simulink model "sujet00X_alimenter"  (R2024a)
settings: Solver=FixedStepDiscrete  StartTime=0.0  StopTime=0.25  FixedStep=Ts  MaxStep=2e-6  EnableMultiTasking=on
PreLoadFcn:
  | assignin('base','Ts',1e-6);
InitFcn:
  | Ts=1e-6;
undefined symbols (not defined in the file): DiscIntNeverNeededParam, sigbuilder_block
libraries: spsUniversalBridgeLib x2, spsCurrentMeasurementLib x2, spsDCVoltageSourceLib x1, spsStepperMotorLib x1, spspowerguiLib x1

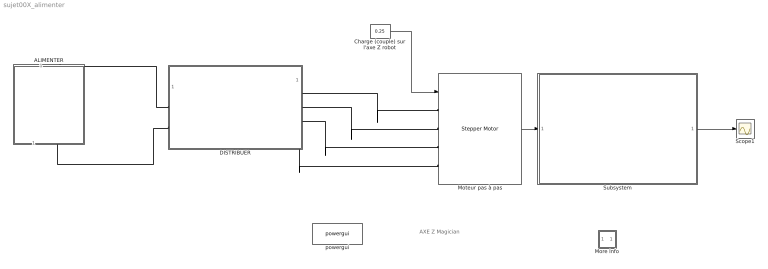
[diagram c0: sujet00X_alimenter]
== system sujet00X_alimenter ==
  note: AXE Z Magician
  ALIMENTER : Subsystem
  Charge (couple) sur l'axe Z robot : Constant  Value=0.25
  DISTRIBUER : Subsystem
  More Info : Subsystem
  Moteur pas à pas : spsStepperMotorLib/Stepper Motor  MotorType=Permanent-magnet / Hybrid  NumberOfPhases_1=2  NumberOfPhases_2=3  PresetModel_1=<empty>  PresetModel_2=<empty>  L=3e-3  Lmax=10e-3  Lmin=2e-3  R=2.1  Step_angle=1.8  Psim=0.005  Tdm=0.002  J=1.2e-7  B=1e-7*1000  w0=0  pos0=0  TsPowergui=0  TsBlock=-1
  Scope1 : Scope
  Subsystem : Subsystem
  powergui : spspowerguiLib/powergui  SimulationMode=Discrete  SampleTime=Ts  frequency=60  Iterations=50  frequencyindice=0  Pbase=100e6  ErrMax=1e-4  UnitsV=kV  UnitsW=MW  buscounter=0  FunctionMessages=off  echomessages=off  EnableUseOfTLC=off  CurrentSourceSwitches=off  DisableSnubberDevices=off  DisableRonSwitches=off  DisableVfSwitches=off  DisplayEquations=off  AutomaticDiscreteSolvers=off  SolverType=Tustin/Backward Euler (TBE)  Interpol=off  ExternalGateDelay=off  methode=off  Ts=0  x0status=blocks  SPID=off  SwTol=0  HookPort=off  NonlinearTolerance=1e-4  nMaxIteration=100  ContinueOnMaxIteration=off  RestoreLinks=warning  ResistiveCurrentMeasurement=off  Frange=[0:2:500]  Ylog=off  Xlog=on  ShowGrid=off  save=off  variable=ZData  structure=0  ZoomFFT=on  StartTime=0.0  cycles=1  DisplayStyle=1  fundamental=60  FreqAxis=off  MaxFrequency=1000  frequencyindicesteady=1  RmsSteady=1  display=off
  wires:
  Charge (couple) sur l'axe Z robot/1 -> Moteur pas à pas/1
  Moteur pas à pas/1 -> Subsystem/1(In1)
  Subsystem/1(Theta (degrees)) -> Scope1/1
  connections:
  DISTRIBUER/RConn1 -- Moteur pas à pas/LConn1
  ALIMENTER/RConn1 -- DISTRIBUER/LConn1
  DISTRIBUER/RConn2 -- Moteur pas à pas/LConn2
  DISTRIBUER/RConn3 -- Moteur pas à pas/LConn3
  DISTRIBUER/RConn4 -- Moteur pas à pas/LConn4
  DISTRIBUER/LConn2 -- ALIMENTER/LConn1

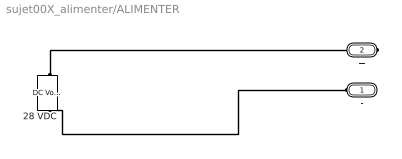
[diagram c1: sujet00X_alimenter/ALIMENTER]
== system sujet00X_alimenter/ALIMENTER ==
  28 VDC : spsDCVoltageSourceLib/DC Voltage Source  Amplitude=25.2  Measurements=None
  - : PMIOPort  Side=Left
  + : PMIOPort  Port=2  Side=Right
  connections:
  -/RConn1 -- 28 VDC/LConn1
  28 VDC/RConn1 -- +/RConn1

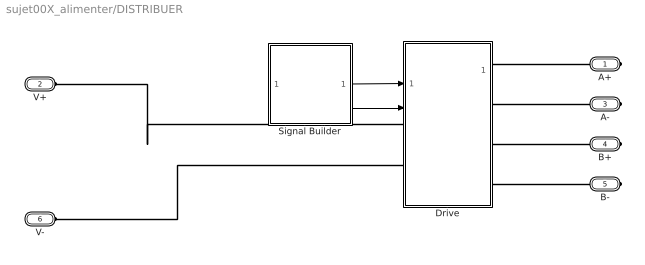
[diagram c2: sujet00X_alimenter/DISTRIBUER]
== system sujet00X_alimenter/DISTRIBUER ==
  Drive : Subsystem  mask{Iref=2, step=1200, Ts=Ts}
      mask prompts: Iref "Phase current (A)"; step "Stepping rate (step/s)"; Ts "Sampling time (s)"
      mask init:
      | Nstep=round(1/step/Ts);
  Signal Builder : Subsystem  Tag=STV Subsys  LoadFcn=sigbuilder_block('load',[90.75 199.5 600 363.75 ]);  StartFcn=sigbuilder_block('start');  StopFcn=sigbuilder_block('stop');  ClipboardFcn=sigbuilder_block('clipboard');  mask(Sigbuilder block){tuvar=[0:10]}
      mask help: Sigbuilder GUI
      mask init:
      | if ~strcmp(get_param(bdroot(gcbh),'SimulationStatus'),'stopped') tuvar = sigbuilder_block('maskInit'); end
  A+ : PMIOPort  Side=Right
  V+ : PMIOPort  Port=2  Side=Left
  A- : PMIOPort  Port=3  Side=Right
  B+ : PMIOPort  Port=4  Side=Right
  B- : PMIOPort  Port=5  Side=Right
  V- : PMIOPort  Port=6  Side=Left
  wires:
  Signal Builder/1(STEP) -> Drive/1(STEP)
  Signal Builder/2(DIR) -> Drive/2(DIR)
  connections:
  Drive/LConn2 -- V-/RConn1
  Drive/RConn4 -- B-/RConn1
  Drive/RConn1 -- A+/RConn1
  Drive/RConn2 -- A-/RConn1
  V+/RConn1 -- Drive/LConn1
  Drive/RConn3 -- B+/RConn1

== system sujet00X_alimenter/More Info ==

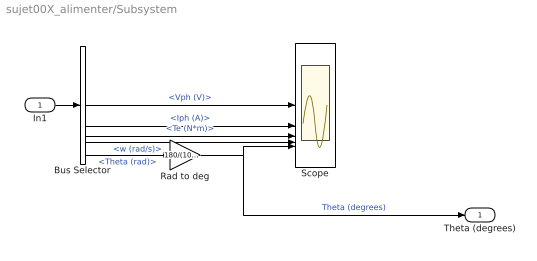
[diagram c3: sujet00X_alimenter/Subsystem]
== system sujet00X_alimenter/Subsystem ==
  In1 : Inport
  Bus Selector : BusSelector  OutputSignals=Vph (V),Iph (A),Te (N*m),w (rad/s),Theta (rad)
  Rad to deg : Gain  Gain=180/(10*pi)
  Scope : Scope  NumInputPorts=5
  Theta (degrees) : Outport
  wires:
  Rad to deg/1 -> Theta (degrees)/1, Scope/5  "Theta (degrees)"
  Bus Selector/2 -> Scope/2  "<Iph (A)>"
  Bus Selector/4 -> Scope/4  "<w (rad/s)>"
  Bus Selector/3 -> Scope/3  "<Te (N*m)>"
  Bus Selector/5 -> Rad to deg/1  "<Theta (rad)>"
  Bus Selector/1 -> Scope/1  "<Vph (V)>"
  In1/1 -> Bus Selector/1

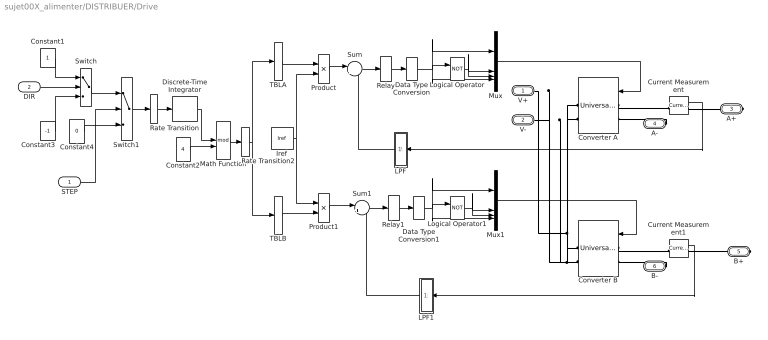
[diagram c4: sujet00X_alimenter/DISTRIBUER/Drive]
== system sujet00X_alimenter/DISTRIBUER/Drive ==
  STEP : Inport
  DIR : Inport  Port=2
  Constant1 : Constant  SampleTime=Ts
  Constant2 : Constant  Value=4  SampleTime=Nstep*Ts
  Constant3 : Constant  Value=-1  SampleTime=Ts
  Constant4 : Constant  Value=0  SampleTime=Ts
  Converter A : spsUniversalBridgeLib/Universal Bridge  Arms=2  SnubberResistance=10000  SnubberCapacitance=inf  Device=MOSFET / Diodes  Ron=1e-3*10  Lon=0  ForwardVoltages="[  0  0  ]"  ForwardVoltage=0  GTOparameters=[ 10e-6 , 20e-6 ]  IGBTparameters=[ 0.5e-6 , 0.5e-6 ]  Measurements=None  Measurements_2=None  converterType=Rectifier
  Converter B : spsUniversalBridgeLib/Universal Bridge  Arms=2  SnubberResistance=10000  SnubberCapacitance=inf  Device=MOSFET / Diodes  Ron=1e-3*10  Lon=0  ForwardVoltages="[  0  0  ]"  ForwardVoltage=0  GTOparameters=[ 10e-6 , 20e-6 ]  IGBTparameters=[ 0.5e-6 , 0.5e-6 ]  Measurements=None  Measurements_2=None  converterType=Rectifier
  Current Measurement : spsCurrentMeasurementLib/Current Measurement  PhasorSimulation=off  OutputType=Complex  PSBequivalent=0
  Current Measurement1 : spsCurrentMeasurementLib/Current Measurement  PhasorSimulation=off  OutputType=Complex  PSBequivalent=0
  Data Type Conversion : DataTypeConversion
  Data Type Conversion1 : DataTypeConversion
  Discrete-Time Integrator : DiscreteIntegrator  IntegratorMethod=Accumulation: Forward Euler  SampleTime=Nstep*Ts  ICPrevOutput=DiscIntNeverNeededParam  ICPrevScaledInput=DiscIntNeverNeededParam
  Iref : Constant  Value=Iref  SampleTime=Ts
  LPF : Subsystem  mask{fc=10000, Ts=Ts}
      mask prompts: fc "Cut-off frequency (Hz)"; Ts "Sampling time (s)"
      mask init:
      | % fa=tf(1,[1/2/pi/fc 1]);
      | % fn=c2d(fa,Ts);
      | % [NN,DD]=tfdata(fn,'v')
      | 
      | NN = [ 0,0.0609];
      | DD = [1.0000,-0.9391];
  LPF1 : Subsystem  mask{fc=10000, Ts=Ts}
      mask prompts: fc "Cut-off frequency (Hz)"; Ts "Sampling time (s)"
      mask init:
      | % fa=tf(1,[1/2/pi/fc 1]);
      | % fn=c2d(fa,Ts);
      | % [NN,DD]=tfdata(fn,'v')
      | 
      | NN = [ 0,0.0609];
      | DD = [1.0000,-0.9391];
  Logical Operator : Logic  Operator=NOT  AllPortsSameDT=off  OutDataTypeStr=boolean
  Logical Operator1 : Logic  Operator=NOT  AllPortsSameDT=off  OutDataTypeStr=boolean
  Math Function : Math  Operator=mod  SignedPower=on  SampleTime=Nstep*Ts
  Mux : Mux
  Mux1 : Mux
  Product : Product  RndMeth=Zero
  Product1 : Product  RndMeth=Zero
  Rate Transition : RateTransition
  Rate Transition2 : RateTransition
  Relay : Relay  OnSwitchValue=0.01  OffSwitchValue=-0.01
  Relay1 : Relay  OnSwitchValue=0.01  OffSwitchValue=-0.01  OutDataTypeStr=Inherit: Inherit via back propagation
  Sum : Sum  Inputs=|+-
  Sum1 : Sum  Inputs=|+-
  Switch : Switch  Threshold=0.5  ZeroCross=off  SampleTime=Ts
  Switch1 : Switch  Threshold=0.5  ZeroCross=off  SampleTime=Ts
  TBLA : Lookup_n-D  NumberOfTableDimensions=1  BreakpointsForDimension1=[0:3]  BreakpointsForDimension2=[0 571.55 685.8 800.15 914.4 1028.8 1143.1 1257.4 1371.7 1486 1600.3 1714.6 1828.9 1943.2 2057.5 2171.8 2286.1 2400.5 2514.7 2629.1 2743.3 2857.7 2971.9 3086.3 3200.5 3314.9 3429.2]  Table=[1 0 -1 0]  InternalRulePriority=Speed  RndMeth=Simplest
  TBLB : Lookup_n-D  NumberOfTableDimensions=1  BreakpointsForDimension1=[0:3]  BreakpointsForDimension2=[0 571.55 685.8 800.15 914.4 1028.8 1143.1 1257.4 1371.7 1486 1600.3 1714.6 1828.9 1943.2 2057.5 2171.8 2286.1 2400.5 2514.7 2629.1 2743.3 2857.7 2971.9 3086.3 3200.5 3314.9 3429.2]  Table=[0 1 0 -1]  InternalRulePriority=Speed  RndMeth=Simplest
  V+ : PMIOPort  Side=Left
  V- : PMIOPort  Port=2  Side=Left
  A+ : PMIOPort  Port=3  Side=Right
  A- : PMIOPort  Port=4  Side=Right
  B+ : PMIOPort  Port=5  Side=Right
  B- : PMIOPort  Port=6  Side=Right
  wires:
  Constant4/1 -> Switch1/3
  Switch1/1 -> Rate Transition/1
  Switch/1 -> Switch1/1
  STEP/1 -> Switch1/2
  DIR/1 -> Switch/2
  Rate Transition2/1 -> TBLB/1, TBLA/1
  Math Function/1 -> Rate Transition2/1
  Product1/1 -> Sum1/1
  Product/1 -> Sum/1
  Rate Transition/1 -> Discrete-Time Integrator/1
  Constant3/1 -> Switch/3
  Constant1/1 -> Switch/1
  Discrete-Time Integrator/1 -> Math Function/1
  Constant2/1 -> Math Function/2
  Iref/1 -> Product1/1, Product/2
  TBLB/1 -> Product1/2
  TBLA/1 -> Product/1
  LPF1/1(O) -> Sum1/2
  LPF/1(O) -> Sum/2
  Data Type Conversion1/1 -> Mux1/4, Mux1/1, Logical Operator1/1
  Data Type Conversion/1 -> Logical Operator/1, Mux/4, Mux/1
  Current Measurement1/1 -> LPF1/1(I)
  Sum1/1 -> Relay1/1
  Mux1/1 -> Converter B/1
  Logical Operator1/1 -> Mux1/2, Mux1/3
  Relay1/1 -> Data Type Conversion1/1
  Mux/1 -> Converter A/1
  Logical Operator/1 -> Mux/2, Mux/3
  Relay/1 -> Data Type Conversion/1
  Current Measurement/1 -> LPF/1(I)
  Sum/1 -> Relay/1
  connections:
  Converter B/RConn2 -- Converter A/RConn2 -- V-/RConn1
  Converter B/RConn1 -- Converter A/RConn1 -- V+/RConn1
  Current Measurement1/RConn1 -- B+/RConn1
  Converter B/LConn1 -- Current Measurement1/LConn1
  Current Measurement/RConn1 -- A+/RConn1
  Converter A/LConn1 -- Current Measurement/LConn1
  B-/RConn1 -- Converter B/LConn2
  A-/RConn1 -- Converter A/LConn2

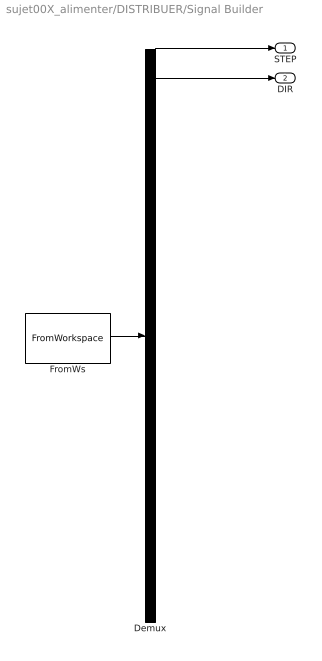
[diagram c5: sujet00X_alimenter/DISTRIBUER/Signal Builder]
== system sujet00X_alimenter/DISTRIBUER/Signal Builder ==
  Demux : Demux  Tag=STV Demux  Outputs=2
  FromWs : FromWorkspace  Tag=STV FromWs  VariableName=tuvar
  STEP : Outport  Tag=STV Outport  VectorParamsAs1DForOutWhenUnconnected=off
  DIR : Outport  Tag=STV Outport  Port=2  VectorParamsAs1DForOutWhenUnconnected=off
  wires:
  FromWs/1 -> Demux/1
  Demux/1 -> STEP/1
  Demux/2 -> DIR/1

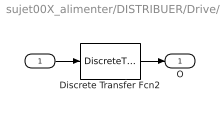
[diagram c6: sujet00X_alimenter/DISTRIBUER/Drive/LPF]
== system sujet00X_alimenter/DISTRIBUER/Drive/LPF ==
  I : Inport
  Discrete Transfer Fcn2 : DiscreteTransferFcn  Numerator=NN  Denominator=DD  SampleTime=Ts
  O : Outport  VectorParamsAs1DForOutWhenUnconnected=off
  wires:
  Discrete Transfer Fcn2/1 -> O/1
  I/1 -> Discrete Transfer Fcn2/1

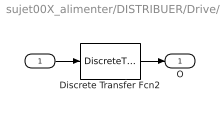
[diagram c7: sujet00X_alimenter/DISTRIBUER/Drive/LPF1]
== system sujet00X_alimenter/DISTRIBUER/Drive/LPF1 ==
  I : Inport
  Discrete Transfer Fcn2 : DiscreteTransferFcn  Numerator=NN  Denominator=DD  SampleTime=Ts
  O : Outport  VectorParamsAs1DForOutWhenUnconnected=off
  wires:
  I/1 -> Discrete Transfer Fcn2/1
  Discrete Transfer Fcn2/1 -> O/1
